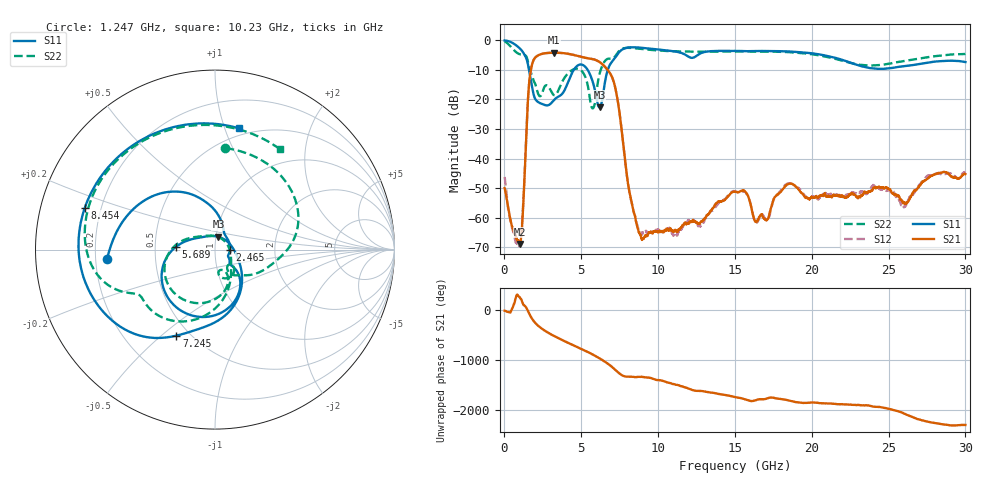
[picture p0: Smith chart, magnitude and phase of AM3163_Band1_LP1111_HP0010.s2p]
!Agilent Technologies,E8364B,MY43040894,A.07.50.67
!Agilent E8364B: A.07.50.67
!Date: Thursday, August 20, 2020 11:57:39
!Correction: S11(Full 2 Port(1,2))
!S21(Full 2 Port(1,2))
!S12(Full 2 Port(1,2))
!S22(Full 2 Port(1,2))
!S2P File: Measurements: S11, S21, S12, S22:
# Hz S  dB  R 50
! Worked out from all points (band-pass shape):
!   3201 points, 10 MHz to 30 GHz, reference 50 ohm
!   highest |S21| = -4.21 dB at 3.234 GHz (marker M1); lowest = -68.8 dB at 1.003 GHz (marker M2)
!   |S21| within 3 dB of the highest: 1.853 GHz to 6.149 GHz (4.296 GHz wide, 107 % of centre)
!   lowest |S11| = -22.6 dB at 6.186 GHz (marker M3), VSWR 1.16, Z = 51.4 + j7.37 ohm
!   |S11| at or under -10 dB: 1.597 GHz to 4.513 GHz (2.916 GHz wide, 95.4 % of centre); 5.413 GHz to 6.725 GHz (1.311 GHz wide, 21.6 % of centre)
!   |S22| runs from -23.0 to -0.4 dB; largest |S21 - S12| = 0.0047
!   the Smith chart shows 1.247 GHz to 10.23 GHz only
!   S11 on the Smith chart (normalised r, x): 1.247 GHz: 0.25, -0.04; 2.465 GHz: 1.18, +0.00; 5.689 GHz: 0.64, +0.02; 7.245 GHz: 0.43, -0.56; 8.454 GHz: 0.14, +0.15; 10.23 GHz: 0.43, +1.12
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1e7  -0.06 -8.7  -49.92 -24.1  -46.15 -49.3  -0.35 -15.4
4.411062e8  -0.66 -57.2  -61.75 -20.3  -62.17 -72.0  -2.33 -95.4
1.003419e9  -2.78 -134.4  -68.78 -120.4  -69.47 138.8  -4.72 144.3
1.247088e9  -4.39 -175.1  -53.01 91.7  -52.64 -13.6  -4.91 84.1
1.687566e9  -12.60 93.5  -11.02 -128.1  -11.02 -128.2  -10.36 -20.3
2.062441e9  -20.26 52.4  -5.56 75.4  -5.57 75.3  -15.80 -56.8
2.465431e9  -21.53 0.2  -4.56 -26.9  -4.57 -26.9  -17.65 -42.2
3.233925e9  -20.13 -35.0  -4.21 -166.0  -4.22 -166.0  -18.55 -76.5
3.955559e9  -16.40 -43.6  -4.42 85.1  -4.44 85.2  -12.30 -79.0
5.014581e9  -8.20 -120.0  -5.65 -64.9  -5.63 -64.7  -10.29 -157.0
5.689356e9  -13.14 176.4  -6.31 -164.3  -6.28 -164.4  -22.76 78.6
6.186066e9  -22.64 74.9  -7.33 110.8  -7.36 110.6  -11.45 -78.4
7.245088e9  -5.60 -114.1  -16.84 -127.5  -16.83 -126.8  -5.16 -154.5
8.454059e9  -2.36 162.2  -58.71 100.0  -58.68 99.0  -2.68 132.4
1.000979e10  -3.11 88.2  -64.82 38.1  -64.20 41.4  -3.45 65.6
1.022534e10  -3.23 79.0  -64.68 29.0  -64.65 21.8  -3.53 57.3
1.5005e10  -3.59 -72.0  -51.19 59.6  -51.01 60.4  -3.79 -92.5
1.639204e10  -3.62 -105.5  -61.19 0.9  -61.37 6.5  -3.79 -126.4
2.000958e10  -4.41 162.5  -53.03 -46.1  -52.76 -55.8  -4.71 135.5
2.274617e10  -7.98 59.7  -52.12 -92.7  -51.59 -100.3  -7.93 20.3
2.500479e10  -9.51 -62.9  -50.28 -170.4  -50.59 -170.9  -7.96 -93.2
3e10  -7.36 104.2  -45.19 -133.9  -44.57 -135.4  -4.64 100.6
